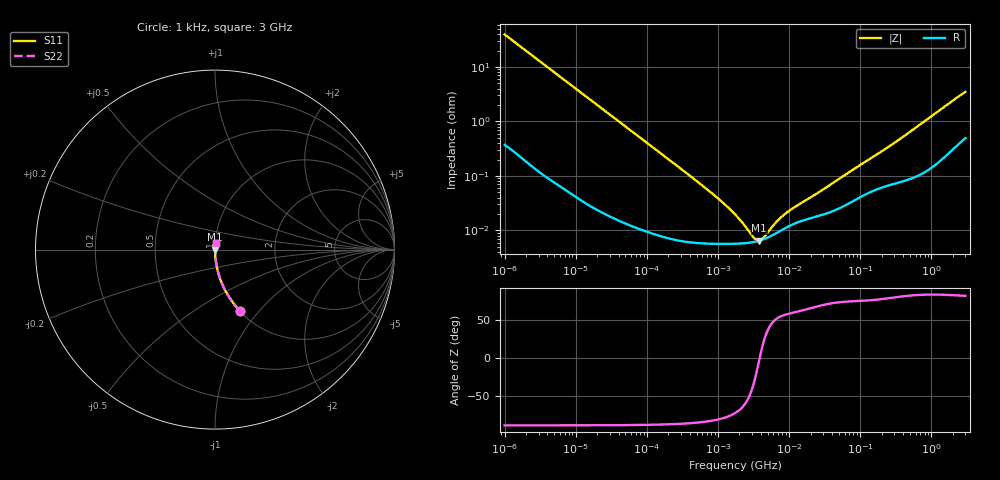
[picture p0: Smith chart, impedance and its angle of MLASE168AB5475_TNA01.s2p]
! MLASE168AB5475_TNA01  S-PARAMETER MODEL  ( Standard Model )
! Model Generated by TAIYO YUDEN Corporation (http://www.ty-top.com)
! Version 1.0
! TAIYO YUDEN Control No. 220601
! Copyright(c) 2010 TAIYO YUDEN CO.,LTD. All Rights Reserved.
! Product Description (link to TY-COMPAS)
! https://ds.yuden.co.jp/TYCOMPAS/or/detail?pn=MLASE168AB5475KTNA01&u=M
! Products Name : Multilayer Ceramic Capacitors
! Characteristics :
!  Capacitance : 4.7 [uF] , Rated Voltage : 16 [V] , TCC : X5R
!  Case Size : 1.6 x 0.8 / 0.063 x 0.031 [mm/inch] , Thickness : 0.8 / 0.031 [mm/inch]
!  (Conditions: Temperature = 25 [degC] , DC Bias Voltage = 0 [V])
! External Node Assignments :
!  1  o---| |---o  2
! GND o---------o GND
! Frequency Range : 1kHz  -  3GHz  [ 401 STEP ]
# MHZ S RI R 50
! Freq[MHz].  S11 Real  S11 Imag  S21 Real  S21 Imag  S12 Real  S12 Imag  S22 Real  S22 Imag
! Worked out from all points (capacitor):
!   401 points, 1 kHz to 3 GHz, reference 50 ohm
!   read as one part in series: C = 4.02 uF near 1.077 kHz
!   lowest |Z| = 6.49 mohm at 3.79 MHz (marker M1)
!   series resonance near 3.856 MHz, so ESL is about 420 pH
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0.001  0.1373 -0.3395  0.8627 0.3395  0.8627 0.3395  0.1373 -0.3395
0.001685  0.0543 -0.222  0.9457 0.222  0.9457 0.222  0.0543 -0.222
0.00306  0.0177 -0.1275  0.9823 0.1275  0.9823 0.1275  0.0177 -0.1275
0.005768  0.00542 -0.0688  0.9946 0.0688  0.9946 0.0688  0.00542 -0.0688
0.01216  0.00143 -0.0329  0.9986 0.0329  0.9986 0.0329  0.00143 -0.0329
0.033275  0.000316 -0.0121  0.9997 0.0121  0.9997 0.0121  0.000316 -0.0121
0.147855  8.77e-05 -0.00275  0.9999 0.00275  0.9999 0.00275  8.77e-05 -0.00275
0.791611  5.73e-05 -0.000496  0.9999 0.000496  0.9999 0.000496  5.73e-05 -0.000496
1.238299  5.67e-05 -0.000297  0.9999 0.000297  0.9999 0.000297  5.67e-05 -0.000297
1.732051  5.7e-05 -0.000189  0.9999 0.000189  0.9999 0.000189  5.7e-05 -0.000189
2.514714  5.88e-05 -9.4e-05  0.9999 9.4e-05  0.9999 9.4e-05  5.88e-05 -9.4e-05
2.709407  5.94e-05 -7.68e-05  0.9999 7.68e-05  0.9999 7.68e-05  5.94e-05 -7.68e-05
2.919173  6.02e-05 -6.01e-05  0.9999 6.01e-05  0.9999 6.01e-05  6.02e-05 -6.01e-05
3.789741  6.48e-05 -3.63e-06  0.9999 3.63e-06  0.9999 3.63e-06  6.48e-05 -3.63e-06
4.919932  7.33e-05 5.12e-05  0.9999 -5.12e-05  0.9999 -5.12e-05  7.33e-05 5.12e-05
5.30084  7.67e-05 6.67e-05  0.9999 -6.67e-05  0.9999 -6.67e-05  7.67e-05 6.67e-05
7.143107  9.49e-05 0.000128  0.9999 -0.000128  0.9999 -0.000128  9.49e-05 0.000128
9.273352  0.000115 0.00018  0.9999 -0.00018  0.9999 -0.00018  0.000115 0.00018
21.06097  0.000171 0.000385  0.9998 -0.000385  0.9998 -0.000385  0.000171 0.000385
256.0921  0.000688 0.00343  0.9993 -0.00343  0.9993 -0.00343  0.000688 0.00343
1917.819  0.00344 0.023  0.9966 -0.023  0.9966 -0.023  0.00344 0.023
3000  0.00611 0.0343  0.9939 -0.0343  0.9939 -0.0343  0.00611 0.0343
